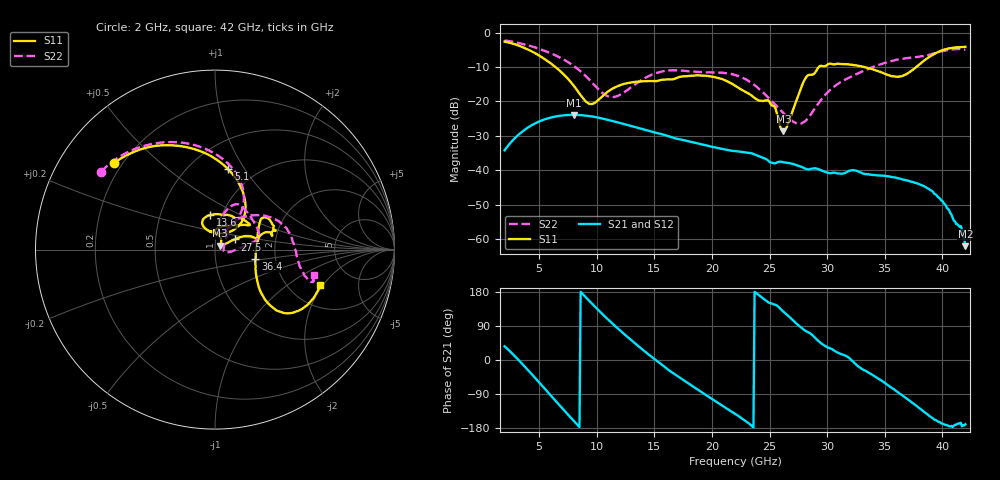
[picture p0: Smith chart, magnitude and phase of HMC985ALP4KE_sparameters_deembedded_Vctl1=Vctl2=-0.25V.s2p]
!s2p File: Measurements: S11, S21, S12, S22
# GHz S dB R 50.0
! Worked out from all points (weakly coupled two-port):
!   401 points, 2 GHz to 42 GHz, reference 50 ohm
!   highest |S21| = -23.89 dB at 8 GHz (marker M1); lowest = -62.0 dB at 42 GHz (marker M2)
!   lowest |S11| = -28.6 dB at 26.2 GHz (marker M3), VSWR 1.08, Z = 53 + j2.37 ohm
!   |S11| at or under -10 dB: 6.414 GHz to 29.27 GHz (22.86 GHz wide, 128 % of centre); 33.23 GHz to 37.73 GHz (4.506 GHz wide, 12.7 % of centre)
!   |S22| runs from -26.5 to -2.3 dB; largest |S21 - S12| = 0.0002
!   S11 on the Smith chart (normalised r, x): 2 GHz: 0.17, +0.36; 5.1 GHz: 0.75, +0.85; 13.6 GHz: 0.88, +0.35; 27.5 GHz: 1.24, +0.14; 36.4 GHz: 1.57, -0.17; 42 GHz: 2.93, -1.90
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2  -2.61 139.1  -34.17 36.2  -34.17 36.2  -2.28 145.6
3.5  -4.14 110.9  -28.83 -9.3  -28.84 -9.2  -3.24 121.8
5.1  -6.88 80.6  -25.66 -62.5  -25.67 -62.5  -4.82 97.4
8  -15.41 45.4  -23.89 -160.6  -23.89 -160.6  -9.67 60.6
8.7  -18.61 54.1  -23.98 176.6  -23.99 176.6  -11.57 55.7
9.6  -20.71 87.8  -24.35 148.2  -24.36 148.2  -14.54 53.9
11.2  -16.62 116.7  -25.53 100.6  -25.53 100.6  -18.70 69.6
13.6  -14.23 98.3  -27.68 36.9  -27.68 36.9  -14.40 77.9
15.4  -13.92 73.4  -29.29 -6.5  -29.30 -6.4  -11.49 68.3
19.4  -12.51 35.5  -32.70 -90.8  -32.70 -90.8  -11.52 34.5
22  -15.37 53.0  -34.40 -141.7  -34.41 -141.6  -12.30 13.9
25  -20.11 95.3  -37.53 150.5  -37.54 150.5  -19.26 -2.2
26.2  -28.61 37.1  -37.63 127.6  -37.64 127.7  -23.38 -13.6
27.5  -18.21 27.5  -38.66 91.6  -38.69 91.7  -26.43 -1.6
28.1  -13.32 19.8  -39.48 77.2  -39.45 77.1  -25.68 19.7
28.7  -12.22 12.1  -39.50 66.2  -39.46 65.9  -23.16 37.0
31.1  -9.12 23.3  -40.93 17.0  -40.94 17.1  -14.52 55.3
35.4  -12.42 12.0  -41.80 -69.2  -41.81 -69.0  -8.42 25.8
36.4  -12.72 -13.1  -42.51 -90.6  -42.50 -91.0  -7.65 17.1
39.6  -5.70 -42.8  -47.65 -162.0  -47.53 -160.7  -5.76 -15.7
41.5  -4.21 -22.9  -56.40 -167.5  -56.54 -167.9  -4.76 -17.6
42  -4.14 -18.8  -62.01 -169.6  -61.43 -168.3  -4.91 -14.7
